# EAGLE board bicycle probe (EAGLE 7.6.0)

Size 73.58 x 63.39 mm. Coordinates in mm from the lower left corner, seen from the top.
Outline: 0,0 56.82,0 56.82,53.33 0,53.33 0,0
Copper layers (1*16): Top 0.035mm / dielectric 1.5mm / Bottom 0.035mm
Design rules "default": minimum track width 10mil, minimum drill 24mil, track to track 8mil, track to pad 8mil, pad to pad 8mil, via to via 8mil, smd to smd 8mil, copper to edge 40mil, drill to drill 8mil, minimum pad ring 10mil, minimum via ring 8mil, stop-mask expansion 4mil, vias tented up to drill 0mil, thermal gap 10mil

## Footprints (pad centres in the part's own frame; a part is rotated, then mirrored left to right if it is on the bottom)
LED5MM = drill 0.813 octagon: A -1.27,0; K 1.27,0
SNR6-D19.0MM = drill 1.3 pad 2: 1 -3.355,3.355; 2 -3.355,-3.355; 3 3.355,3.355; 4 3.355,-3.355; 5 0,4.75; 6 0,-4.75
0207/10 = drill 0.813 octagon: 1 -5.08,0; 2 5.08,0
PHOTORESISTOR-2.54 = drill 1 pad 1.5: P$1 -1.27,0; P$2 1.27,0
ARDUINO_UNO = drill 1.016 pad 1.88: 0 63.5,50.8; 1 60.96,50.8; 2 58.42,50.8; 3 55.88,50.8; 3.3V 35.56,2.54; 4 53.34,50.8; 5 50.8,50.8; 5V 38.1,2.54; 6 48.26,50.8; 7 45.72,50.8; 8 41.656,50.8; 9 39.116,50.8; 10 36.576,50.8; 11 34.036,50.8; 12 31.496,50.8; 13 28.956,50.8; A0 50.8,2.54; A1 53.34,2.54; A2 55.88,2.54; A3 58.42,2.54; A4 60.96,2.54; A5 63.5,2.54; AREF 23.876,50.8; GND 26.416,50.8; GND. 43.18,2.54; GND.. 40.64,2.54; I/OREF 30.48,2.54; N/C 27.94,2.54; RESET 33.02,2.54; SCL 18.796,50.8; SDA 21.336,50.8; VIN 45.72,2.54 | hole 3.2: 66.04,7.62; 66.04,35.56; 15.24,50.8; 13.97,2.54
TO92 = drill 0.813 octagon: 1 1.27,0; 2 0,1.905; 3 -1.27,0
2X4P-2.54-65/35MIL = drill 0.889 pad 1.651 square: 1 -1.27,3.81 | drill 0.889 pad 1.651: 2 -1.27,1.27; 3 -1.27,-1.27; 4 -1.27,-3.81; 5 1.27,-3.81; 6 1.27,-1.27; 7 1.27,1.27; 8 1.27,3.81

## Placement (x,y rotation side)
D1  [LED5MM]  5,22.78 0 top
D2  [LED5MM]  not placed on the board
D3  [LED5MM]  not placed on the board
D4  [LED5MM]  not placed on the board
D5  [LED5MM]  not placed on the board
D6  [LED5MM]  not placed on the board
GAS1  [SNR6-D19.0MM]  not placed on the board
R1  1k‎Ω  [0207/10]  5,35.48 0 top
R2  [PHOTORESISTOR-2.54]  5,60.88 0 top
R3  1k‎Ω  [0207/10]  5,48.18 0 top
R5  1k‎Ω  [0207/10]  not placed on the board
R6  1k‎Ω  [0207/10]  not placed on the board
R8  1k‎Ω  [0207/10]  not placed on the board
R9  1k‎Ω  [0207/10]  not placed on the board
R10  1k‎Ω  [0207/10]  not placed on the board
R11  1k‎Ω  [0207/10]  not placed on the board
U1  [ARDUINO_UNO]  5,10.08 0 top
U2  [TO92]  not placed on the board
U3  [2X4P-2.54-65/35MIL]  not placed on the board
U4  [2X4P-2.54-65/35MIL]  not placed on the board

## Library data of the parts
D1-D6 GAS1 R1-R3 R5 R6 R8-R11 U1-U4 = AUTODESK_CIRCUITS_BREADBOARD

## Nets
N$1: R9.1 R10.1 R11.1 U1.GND.. U2.1
N$2: R2.P$1 R3.1 U1.A0
N$3: D2.A R1.2
N$4: D1.A R6.2
N$5: D1.K U1.8
N$6: D3.K U1.9
N$7: D3.A R5.2
N$8: D2.K U1.7
N$9: GAS1.2 GAS1.4 GAS1.6 R2.P$2 U1.5V
N$10: GAS1.5 R1.1 R3.2 R5.1 R6.1 R8.2 U1.GND.
N$11: GAS1.1 R8.1
N$12: GAS1.3 U1.A1
N$13: U1.3.3V U2.3
N$14: U1.A2 U2.2
N$15: D4.K R9.2
N$16: D4.A U1.4
N$17: D5.K R10.2
N$18: D5.A U1.5
N$19: D6.K R11.2
N$20: D6.A U1.6

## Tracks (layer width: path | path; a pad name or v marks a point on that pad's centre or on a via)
N$1  (4 unrouted)
N$2  (2 unrouted)
N$3  (1 unrouted)
N$4  (1 unrouted)
N$5  (1 unrouted)
N$6  (1 unrouted)
N$7  (1 unrouted)
N$8  (1 unrouted)
N$9  (4 unrouted)
N$10  (6 unrouted)
N$11  (1 unrouted)
N$12  (1 unrouted)
N$13  (1 unrouted)
N$14  (1 unrouted)
N$15  (1 unrouted)
N$16  (1 unrouted)
N$17  (1 unrouted)
N$18  (1 unrouted)
N$19  (1 unrouted)
N$20  (1 unrouted)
